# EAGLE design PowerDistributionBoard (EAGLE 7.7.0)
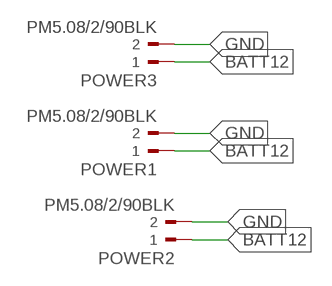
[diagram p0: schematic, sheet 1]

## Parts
POWER1  PM5.08/2/90BLK  [WEIDMULLER_PM5.08_2]
POWER2  PM5.08/2/90BLK  [WEIDMULLER_PM5.08_2]
POWER3  PM5.08/2/90BLK  [WEIDMULLER_PM5.08_2]

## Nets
BATT12: POWER1.1 POWER2.1 POWER3.1
GND: POWER1.2 POWER2.2 POWER3.2

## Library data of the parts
POWER1-POWER3 = WEIDMULLER-PM5.08_2_90BLK:PM5.08/2/90BLK: TERMINAL BLOCK, SIDE ENTRY, 2WAY; MPN: PM5.08/2/90 BLK; OC_FARNELL: 1131855; OC_NEWARK: 26M1980; PACKAGE: TH-R/A; SUPPLIER: WEIDMULLER

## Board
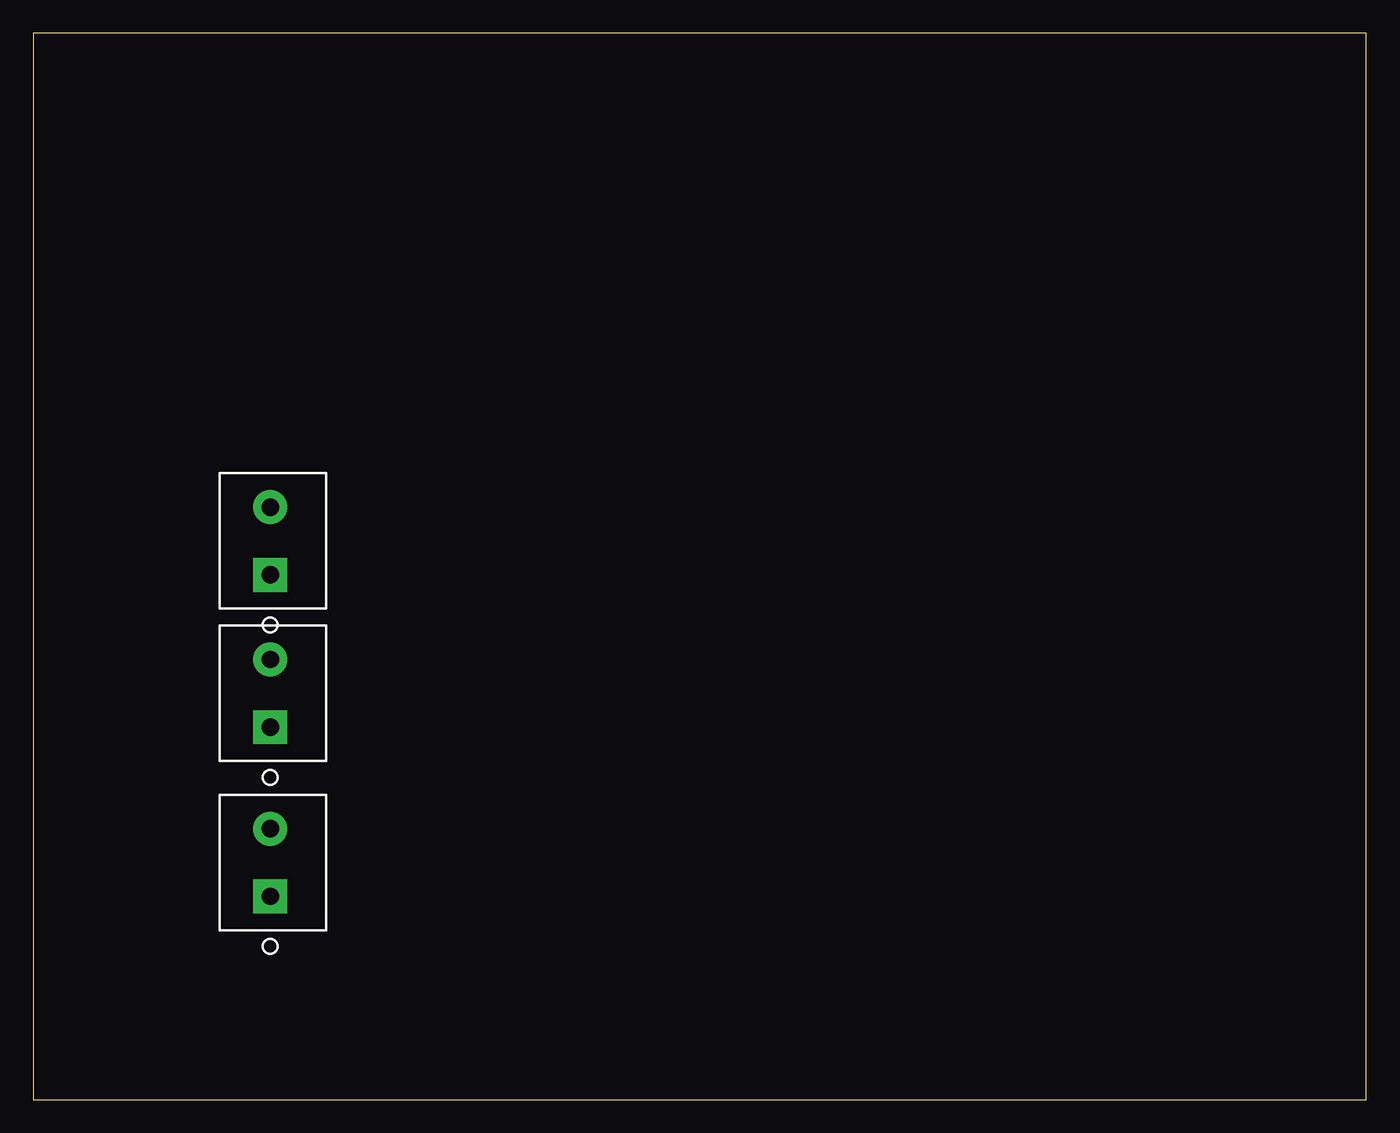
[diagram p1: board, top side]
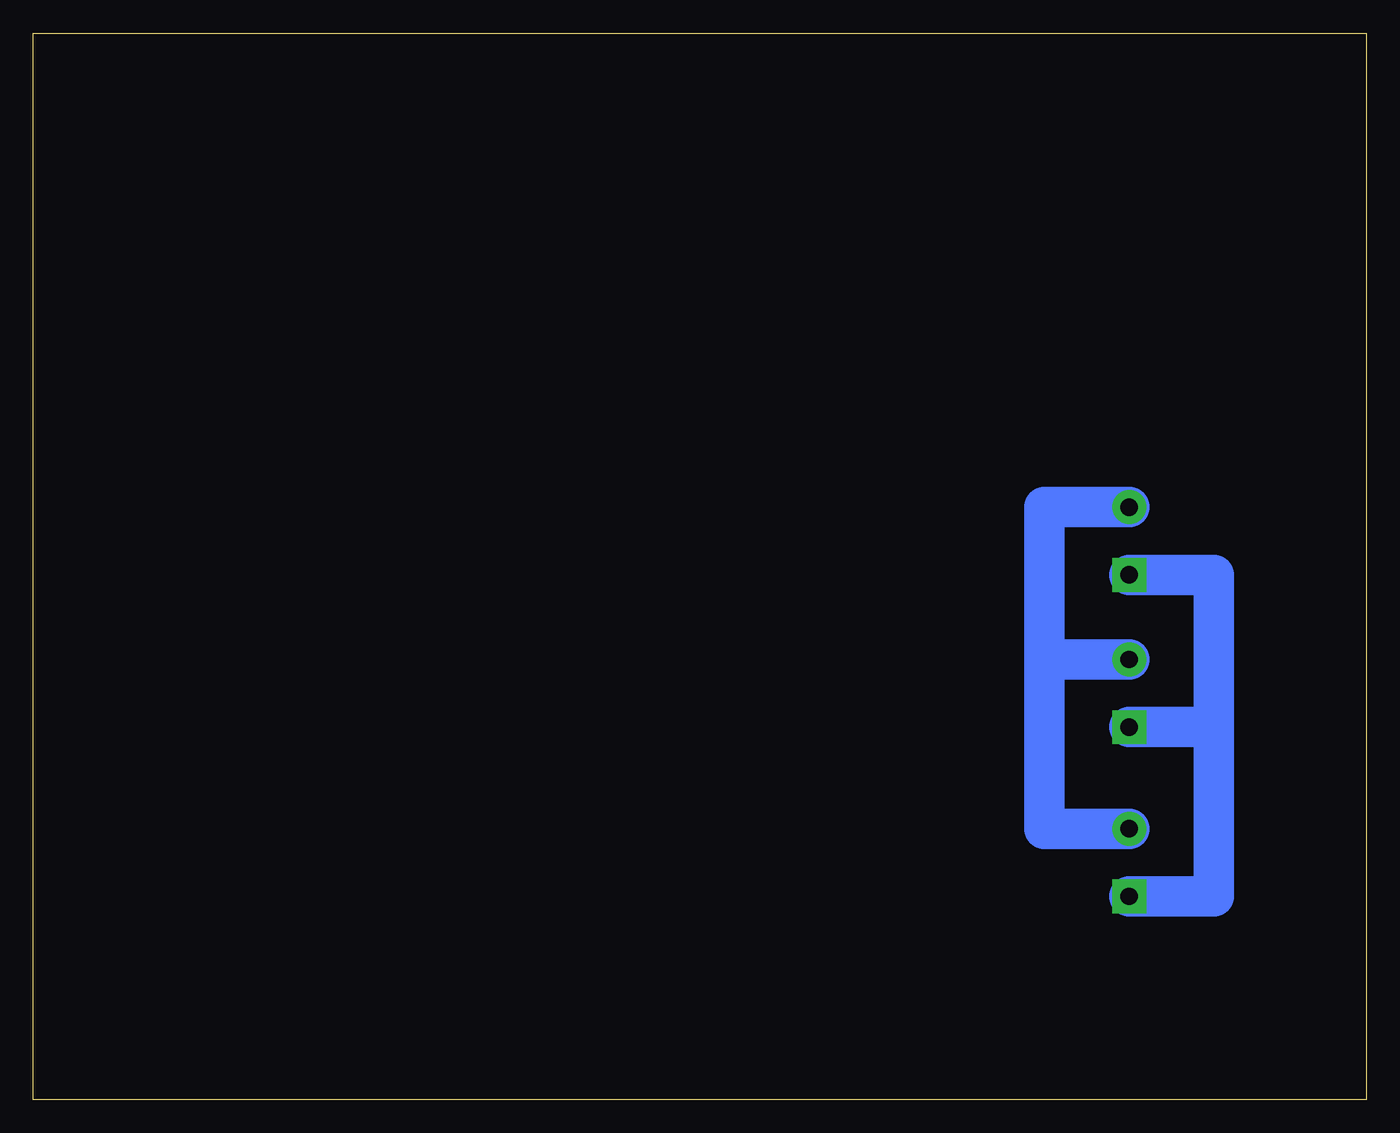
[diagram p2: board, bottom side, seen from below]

Size 100 x 80 mm. Coordinates in mm from the lower left corner, seen from the top.
Outline: 0,0 100,0 100,80 0,80 0,0
Copper layers (1*16): Top 0.035mm / dielectric 1.5mm / Bottom 0.035mm
Design rules "default": minimum track width 10mil, minimum drill 24mil, track to track 8mil, track to pad 8mil, pad to pad 8mil, via to via 8mil, smd to smd 8mil, copper to edge 40mil, drill to drill 8mil, minimum pad ring 10mil, minimum via ring 8mil, stop-mask expansion 4mil, vias tented up to drill 0mil, thermal gap 10mil

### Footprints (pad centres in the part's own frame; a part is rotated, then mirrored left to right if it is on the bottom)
WEIDMULLER_PM5.08_2 = drill 1.3 pad 2.54 square: 1 -2.54,0 | drill 1.3 pad 2.54: 2 2.54,0

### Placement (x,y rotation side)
POWER1  17.78,17.78 90 top
POWER2  17.78,30.48 90 top
POWER3  17.78,41.91 90 top

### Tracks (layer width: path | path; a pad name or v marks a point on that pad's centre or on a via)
BATT12
  Bottom 3.048: 13.97,15.24 POWER1.1 11.43,15.24 11.43,27.94 | POWER3.1 11.43,39.37 11.43,27.94 | 11.43,27.94 POWER2.1
GND
  Bottom 3.048: 21.59,20.32 POWER1.2 24.13,20.32 24.13,33.02 | POWER2.2 24.13,33.02 | POWER3.2 24.13,44.45 24.13,33.02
